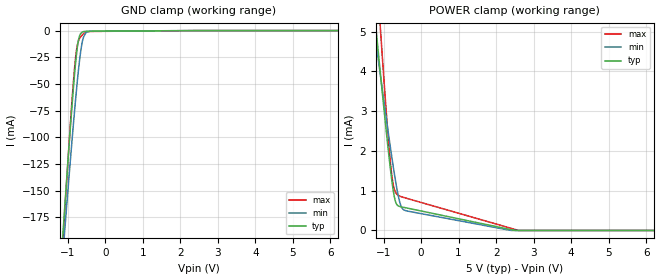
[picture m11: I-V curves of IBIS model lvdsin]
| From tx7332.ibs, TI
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|   lvdsin Model
[Model]   lvdsin
Model_type   Input
Vinl = 1.25
Vinh = 3.75
|   typ   min   max
C_comp   8.865pF   8.197pF   9.198pF
| Where Nom  PVT is Nominal Process, 5.0V, 27C
|   Fast PVT is Strong Process,  5.1V, 0C
|   Slow PVT is Weak Process,   4.9V, 100C
[Voltage Range]   5   4.9   5.1
|Junction Temperature
[Temperature Range]   27   100   0
[Power Clamp Reference]   5   4.9   5.1
[GND Clamp Reference]   0   0   0
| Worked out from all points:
|   GND clamp passes 1 mA (typ) near -0.58 V on its own axis
|   POWER clamp passes 1 mA (typ) near -0.74 V on its own axis
[GND Clamp]
|   Voltage   I(typ)   I(min)   I(max)
-5V       -2.316A    -2.046A    -2.57A
-1.13V    -192.5mA   -210.7mA   -199.5mA
-1.1V     -177mA     -197.2mA   -182.3mA
-1.07V    -161.6mA   -183.8mA   -165.3mA
-905mV    -80.14mA   -111.9mA   -76.06mA
-800mV    -34.63mA   -69.02mA   -29.25mA
-755mV    -19.21mA   -51.97mA   -16.28mA
-710mV    -8.614mA   -36.28mA   -9.538mA
-590mV    -1.102mA   -7.6mA     -3.305mA
-515mV    -658.7uA   -2.156mA   -1.523mA
-365mV    -562.9uA   -540uA     -785.8uA
10V       0A         0A         0A
[POWER Clamp]
|   Voltage   I(typ)   I(min)   I(max)
-5V       43.22mA    32.49mA    63.14mA
-1.25V    5.551mA    5.077mA    7.431mA
-1.13V    4.39mA     4.227mA    5.726mA
-1.1V     4.104mA    4.017mA    5.305mA
-1.055V   3.676mA    3.702mA    4.681mA
-845mV    1.778mA    2.271mA    1.998mA
-740mV    998.1uA    1.599mA    1.141mA
-665mV    685.6uA    1.161mA    936.5uA
-575mV    605.8uA    737.7uA    866.8uA
-440mV    576.4uA    508.5uA    823.7uA
2.59V     0A         0A         2.458uA
10V       0A         0A         0A
